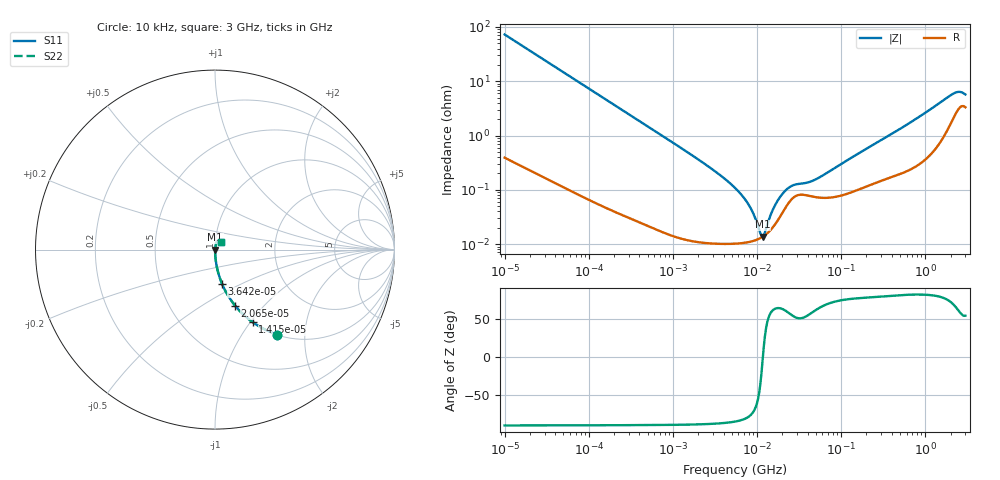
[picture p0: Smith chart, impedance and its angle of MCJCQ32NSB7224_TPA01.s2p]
! MCJCQ32NSB7224_TPA01  S-PARAMETER MODEL  ( Standard Model )
! Model Generated by TAIYO YUDEN Corporation (http://www.ty-top.com)
! Version 1.0
! TAIYO YUDEN Control No. 220601
! Copyright(c) 2015 TAIYO YUDEN CO.,LTD. All Rights Reserved.
! Product Description (link to TY-COMPAS)
! https://ds.yuden.co.jp/TYCOMPAS/or/detail?pn=MCJCQ32NSB7224KTPA01&u=M
! Products Name : Multilayer Ceramic Capacitors
! Characteristics :
!  Capacitance : 0.22 [uF] , Rated Voltage : 250 [V] , TCC : X7R
!  Case Size : 3.2 x 2.5 / 0.126 x 0.098 [mm/inch] , Thickness : 1.9 / 0.075 [mm/inch]
!  (Conditions: Temperature = 25 [degC] , DC Bias Voltage = 0 [V])
! External Node Assignments :
!  1  o---| |---o  2
! GND o---------o GND
! Frequency Range : 10kHz  -  3GHz  [ 401 STEP ]
# MHZ S RI R 50
! Freq[MHz].  S11 Real  S11 Imag  S21 Real  S21 Imag  S12 Real  S12 Imag  S22 Real  S22 Imag
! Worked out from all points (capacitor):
!   401 points, 10 kHz to 3 GHz, reference 50 ohm
!   read as one part in series: C = 219 nF near 10.65 kHz
!   lowest |Z| = 13.6 mohm at 11.67 MHz (marker M1)
!   series resonance near 11.74 MHz, so ESL is about 840 pH
!   S11 on the Smith chart (normalised r, x): 10 kHz: 1.01, -1.45; 14.15 kHz: 1.01, -1.03; 20.65 kHz: 1.00, -0.71; 36.42 kHz: 1.00, -0.40; 3 GHz: 1.07, +0.09
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0.01  0.3466 -0.4732  0.6534 0.4732  0.6534 0.4732  0.3466 -0.4732
0.014146  0.2107 -0.4049  0.7893 0.4049  0.7893 0.4049  0.2107 -0.4049
0.020651  0.1123 -0.3126  0.8877 0.3126  0.8877 0.3126  0.1123 -0.3126
0.036425  0.0399 -0.1923  0.9601 0.1923  0.9601 0.1923  0.0399 -0.1923
0.082683  0.00854 -0.0879  0.9915 0.0879  0.9915 0.0879  0.00854 -0.0879
0.683653  0.000293 -0.0108  0.9997 0.0108  0.9997 0.0108  0.000293 -0.0108
2.737278  0.00011 -0.00258  0.9999 0.00258  0.9999 0.00258  0.00011 -0.00258
5.477226  0.000103 -0.00108  0.9999 0.00108  0.9999 0.00108  0.000103 -0.00108
7.996027  0.000109 -0.000513  0.9999 0.000513  0.9999 0.000513  0.000109 -0.000513
9.361346  0.000116 -0.0003  0.9999 0.0003  0.9999 0.0003  0.000116 -0.0003
10.95979  0.000129 -9.14e-05  0.9999 9.14e-05  0.9999 9.14e-05  0.000129 -9.14e-05
11.67315  0.000136 -7.35e-06  0.9999 7.35e-06  0.9999 7.35e-06  0.000136 -7.35e-06
12.43293  0.000146 7.75e-05  0.9999 -7.75e-05  0.9999 -7.75e-05  0.000146 7.75e-05
14.55585  0.000183 0.000296  0.9998 -0.000296  0.9998 -0.000296  0.000183 0.000296
15.99985  0.000219 0.000431  0.9998 -0.000431  0.9998 -0.000431  0.000219 0.000431
21.24962  0.000438 0.000821  0.9996 -0.000821  0.9996 -0.000821  0.000438 0.000821
27.34599  0.000726 0.000983  0.9993 -0.000983  0.9993 -0.000983  0.000726 0.000983
45.28751  0.000753 0.00124  0.9992 -0.00124  0.9992 -0.00124  0.000753 0.00124
374.4521  0.00175 0.0099  0.9983 -0.0099  0.9983 -0.0099  0.00175 0.0099
2120.803  0.0221 0.0525  0.9779 -0.0525  0.9779 -0.0525  0.0221 0.0525
2482.93  0.0325 0.0525  0.9675 -0.0525  0.9675 -0.0525  0.0325 0.0525
3000  0.034 0.0434  0.966 -0.0434  0.966 -0.0434  0.034 0.0434
